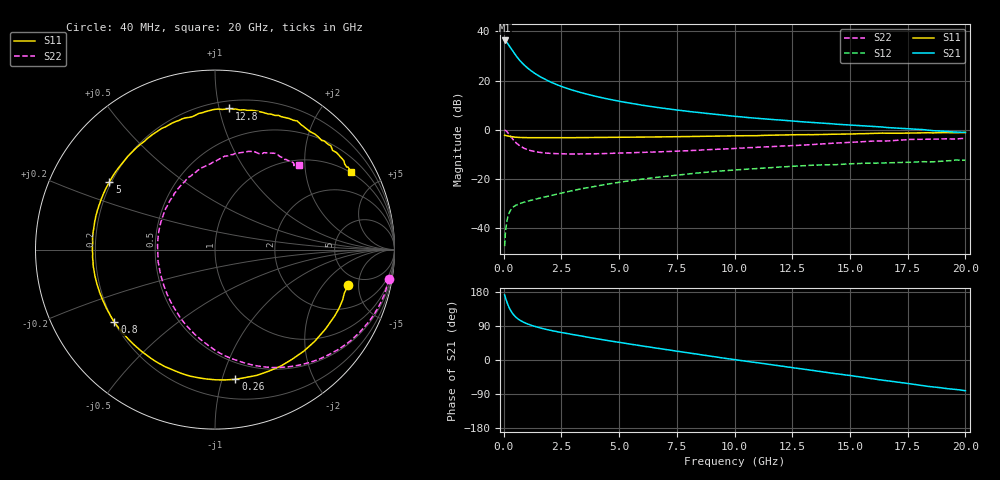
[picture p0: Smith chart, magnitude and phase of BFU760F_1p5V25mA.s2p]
! Filename:  P:\Prog\Test\Noise\ATS_data\Testdata_Net\Split files Spar\BFU760F_2W_C1_Bias6_1.5V_5mA_60mA_D.s2p
! Date/Time: Mon 06/Feb/2012 15:07:37
! BFU760_2W_C1_Bias6_1.5V_5mA_60mA_R.s2p
! MDIF S-parameter v. bias file
! BFU760_2W_C1_1.5V_5mA_60mA
! Date/time Fri Mar 18 11:09:37 2011
! VAR V_out= 1.4999
! VAR I_out= 25.0150
! VAR V_in= 0.7953
! VAR I_in= 0.0799
! Device data file deembeded for feedlines and parallel
! Original file: \Split files Spar\BFU760_2W_C1_Bias6_1.5V_5mA_60mA_R.s2p
! Feed-files: PR003V01_101208_Feed1.s2p, PR003V01_101208_Feed2.s2p
! Parallel-file: PR003V01_101208_Par.s2p
# MHz S MA R 50
!  Freq-MHz  S11-mag  S11-arg  S21-mag  S21-arg  S12-mag  S12-arg  S22-mag  S22-arg
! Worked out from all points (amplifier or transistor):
!   167 points, 40 MHz to 20 GHz, reference 50 ohm
!   highest |S21| = 36.3 dB at 40 MHz (marker M1)
!   |S21| within 3 dB of that: start of sweep to 299 MHz
!   unconditionally stable (mu >= 1): 3.992 GHz to 14.88 GHz
!   at 550 MHz: K = 0.29, MSG = 30.3 dB, |S12| = -30.7 dB
!   at 4.2 GHz: K = 1.01, MAG = 17.3 dB, |S12| = -22.7 dB
!   at 20 GHz: K = 0.92, MSG = 5.7 dB, |S12| = -12.4 dB
!   S11 on the Smith chart (normalised r, x): 40 MHz: 3.94, -3.76; 260 MHz: 0.36, -1.11; 800 MHz: 0.20, -0.31; 5 GHz: 0.19, +0.28; 12.8 GHz: 0.26, +1.07; 20 GHz: 0.96, +3.53
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40  0.7687 -14.7  65.58 171.9  0.004234 83.4  0.9835 -9.6
50  0.7604 -18.6  65.24 169.3  0.004901 79.9  0.9792 -12.4
90  0.759 -32.5  63.24 161.7  0.009232 75.5  0.9562 -22.4
140  0.7517 -48.8  59.72 152.8  0.01365 68.2  0.9091 -34.2
200  0.7406 -66.2  54.63 143.4  0.01796 60.6  0.8407 -46.8
260  0.7316 -81.1  49.63 135.4  0.02121 54.8  0.7715 -57.8
300  0.7256 -89.7  46.34 130.9  0.02299 51.5  0.7291 -64.4
380  0.7155 -104.5  40.74 123.2  0.02563 46.5  0.6506 -75.7
480  0.7052 -118.1  34.68 115.9  0.028 42.3  0.5764 -87.5
600  0.696 -130.3  29.18 109.3  0.02994 39.3  0.5085 -98.9
800  0.6915 -144.2  22.81 101.6  0.03245 37.1  0.4392 -113.7
1200  0.6852 -160.8  15.66 91.5  0.03657 36.9  0.3712 -134.2
1700  0.6841 -173.1  11.17 82.9  0.04188 38.6  0.3381 -150.9
2400  0.6841 175.8  7.907 73.7  0.04981 40.4  0.3237 -166.6
3400  0.6895 163.4  5.601 62.7  0.06278 40.5  0.3208 178.0
5000  0.6991 147.3  3.795 46.5  0.08463 36.6  0.3316 159.0
6800  0.7125 131.5  2.776 29.7  0.1092 28.8  0.3541 141.7
10200  0.751 104.1  1.837 -0.7  0.153 9.6  0.4201 112.8
12800  0.7902 84.3  1.465 -22.5  0.183 -6.6  0.4799 92.7
13400  0.7899 79.9  1.395 -27.6  0.1888 -11.2  0.4986 88.5
16800  0.8452 54.1  1.089 -56.3  0.212 -33.0  0.5959 63.9
20000  0.8741 29.6  0.8813 -81.1  0.2386 -54.4  0.6632 45.3
